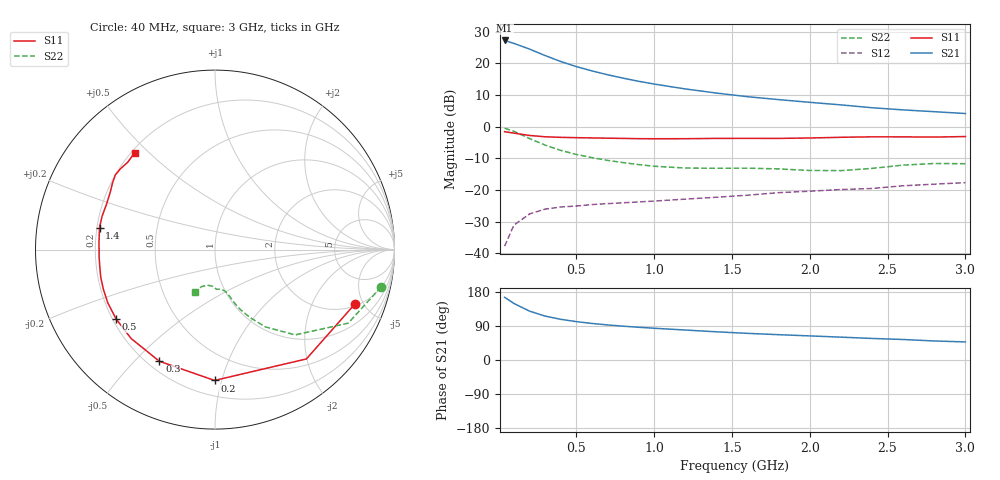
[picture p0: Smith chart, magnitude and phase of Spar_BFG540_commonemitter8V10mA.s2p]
! Filename:  BFG540H.S2P  Version:  3.0
! NXP part #: BFG540  Date: Feb 1992
! Bias condition: Vce=8V, Ic=10mA
! IN LINE PINNING: same data as with cross emitter pinning.
#  MHz  S  MA  R  50
! Freq  S11  S21  S12  S22  !GUM [dB]
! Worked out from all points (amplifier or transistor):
!   21 points, 40 MHz to 3 GHz, reference 50 ohm
!   highest |S21| = 27.3 dB at 40 MHz (marker M1)
!   |S21| within 3 dB of that: start of sweep to 213.5 MHz
!   unconditionally stable (mu >= 1): 1.252 GHz to end of sweep
!   at 300 MHz: K = 0.31, MSG = 24.3 dB, |S12| = -26.0 dB
!   at 1 GHz: K = 0.88, MSG = 18.5 dB, |S12| = -23.5 dB
!   at 3 GHz: K = 1.23, MAG = 8.0 dB, |S12| = -17.7 dB
!   lowest NFmin = 1.30 dB at 900 MHz
!   S11 on the Smith chart (normalised r, x): 40 MHz: 2.16, -4.34; 200 MHz: 0.30, -0.95; 300 MHz: 0.25, -0.59; 500 MHz: 0.21, -0.30; 1.4 GHz: 0.21, +0.09; 3 GHz: 0.21, +0.45
40  0.837 -21.1  23.1 165.5  0.013 77.7  0.949 -12.6
100  0.794 -50.1  20.74 149.2  0.028 63.4  0.848 -28.9
200  0.729 -90.2  16.88 128.9  0.042 48.5  0.652 -46.8
300  0.695 -116.5  13.35 115.9  0.05 41.2  0.514 -56.9
400  0.681 -133.3  10.75 107.4  0.054 37.8  0.424 -62.9
500  0.673 -145.0  8.943 101.3  0.056 37.0  0.366 -66.8
600  0.667 -153.6  7.64 96.5  0.059 37.2  0.326 -69.4
700  0.66 -160.5  6.649 92.6  0.061 37.8  0.295 -71.2
800  0.655 -166.3  5.872 89.3  0.063 38.6  0.272 -72.7
900  0.649 -171.4  5.24 86.4  0.065 40.0  0.253 -74.4
1000  0.647 -176.3  4.732 83.8  0.067 41.5  0.238 -76.4
1200  0.648 175.5  3.964 79.1  0.072 44.3  0.223 -81.4
1400  0.655 169.2  3.412 74.4  0.077 46.4  0.221 -85.8
1600  0.656 163.4  2.987 70.3  0.083 49.8  0.222 -87.8
1800  0.655 157.6  2.686 66.8  0.091 51.4  0.216 -89.4
2000  0.665 151.4  2.434 63.6  0.096 53.8  0.204 -94.2
2200  0.682 146.7  2.218 60.3  0.102 55.1  0.203 -102.6
2400  0.694 143.1  1.999 56.9  0.106 57.1  0.22 -110.2
2600  0.693 139.5  1.848 54.1  0.117 57.8  0.248 -113.6
2800  0.688 135.0  1.731 50.2  0.124 57.1  0.263 -114.0
3000  0.701 129.7  1.619 47.7  0.131 58.9  0.261 -115.5
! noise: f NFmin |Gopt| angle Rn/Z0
900  1.3  0.284  125  0.13
1000  1.4  0.29  134  0.12
2000  2.1  0.505  -167  0.11
